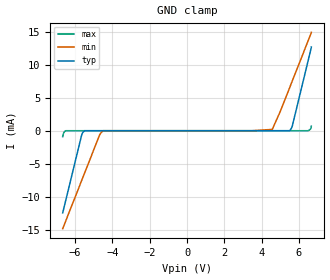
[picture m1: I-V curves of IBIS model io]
|Texas Instruments Incorporated
| TPD1E0B04 1-Channel ESD Protection Diode for USB Type-C and Antenna Protection
| Marketing part#   Digital Voltage Range   Package-type   #pins
| TPD1E0B04DPLR   0.0V-6.6V   X2SON   2
[IBIS Ver]   4.1
[File name]   tpd1e0b04.ibs
[File Rev]   2.0
[Date]   06/16/2016
[Source]
| Texas Instruments Incorporated.
| Analog-eLab Design Center, HPA
| 12500 TI Blvd
| Dallas, TX -75243
[Notes]   Revision History:
| Rev 1.0: 06/10/2016
| - Initial version of the model
| - Model generated from bench data
| - Model matched to SPICE simulation
| - C_comp although listed in numerical order of value are
|   obtained from varying PVT conditions. For PVT conditions for
|   each specific value refer the buffer description under
|   respective [Model]. IBIS model user is responsible for using
|   appropriate C_comp to simulate for Signal Integrity.
[Disclaimer]
| This model is designed as an aid for customers of Texas Instruments.
| TI and its licensors and suppliers make no warranties, either expressed
| or implied, with respect to this  model, including the warranties of
| merchantability or fitness for a particular purpose. The model is
| provided solely on an "as is" basis. The entire risk as to its quality
| and performance is with the customer.
[Copyright]
(C) Copyright 2016 Texas Instruments Incorporated.All rights reserved.
|   TPD1E0B04DPL
[Component]   TPD1E0B04DPL
[Manufacturer]   TI
[Package]   |2 X2SON - DPL package
|   typ   min   max
R_pkg   1.000e-200   1.000e-200   1.000e-200
L_pkg   1.000e-200   1.000e-200   1.000e-200
C_pkg   1.000e-200   1.000e-200   1.000e-200
[Pin]  signal_name   model_name   R_pin   L_pin   C_pin
1   1   io   4.000E-02  3.000E-10  1.000E-14
2   2   gnd   1.000e-200 1.000e-200 1.000e-200
|   TPD1E0B04DPY
[Component]   TPD1E0B04DPY
[Manufacturer]   TI
[Package]   |2 X1SON - DPY package
|   typ   min   max
R_pkg   1.000e-200   1.000e-200   1.000e-200
L_pkg   1.000e-200   1.000e-200   1.000e-200
C_pkg   1.000e-200   1.000e-200   1.000e-200
[Pin]  signal_name   model_name   R_pin   L_pin   C_pin
1   1   io   4.000E-02   6.000E-10   2.000E-14
2   2   gnd   1.000e-200  1.000e-200  1.000e-200
| Models and submodels in the file (1): io (Terminator)
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|   io Model
[Model]   io
Model_type   Terminator
|   typ   min   max
C_comp   1.313E-13   1.125E-13   1.500E-13
| Where nom  PVT is Nominal Process, 6.67V, 25C
|   Fast PVT is Strong Process,  7.0V, -40C
|   Slow PVT is Weak Process,   6.0V, 125C
[Voltage Range]   6.67   6.0   7.0
|Ambient Temperature   25   125   -40
|Junction Temperature
[Temperature Range]   25   125   -40
[Power Clamp Reference]   6.67   6.0   7.0
[GND Clamp Reference]   0   0   0
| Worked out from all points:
|   GND clamp passes 1 mA (typ) near -5.68 V on its own axis
[GND Clamp]
|   Voltage   I(typ)   I(min)   I(max)
-6.67V    -12.43mA   -14.81mA   -900.1uA
-6.612V   -11.76mA   -14.4mA    -300.1uA
-6.5V     -10.46mA   -13.59mA   -616.8pA
-5.667V   -800.1uA   -7.629mA   -330.4pA
-5.5V     -605.2pA   -6.436mA   -306.8pA
-4.697V   -392.2pA   -700.1uA   -272.8pA
-4.495V   -214.8pA   -127.3nA   -270.7pA
4.576V    456.1pA    200.1uA    233.9pA
5.5V      840.7pA    6.458mA    341.1pA
5.657V    800.1uA    7.58mA     359.2pA
6.5V      10.6mA     13.61mA    853.9pA
6.67V     12.66mA    14.87mA    700.1uA
[Power Clamp]
|   Voltage   I(typ)   I(min)   I(max)
-6.67V    0A         0A         0A
0V        0A         0A         0A
6.67V     0A         0A         0A
